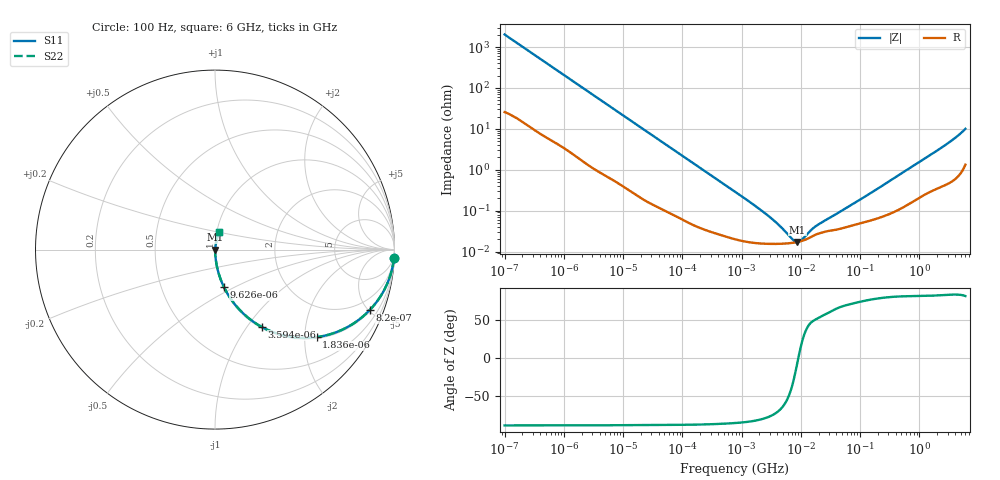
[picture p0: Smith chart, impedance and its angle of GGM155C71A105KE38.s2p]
!Murata Part Number: GGM155C71A105KE38
!These Parameters are Measured in Series Mode Connection
!Data Generated on Jun 19, 2026
!  o--ll--o
!Port1  Port2
!  o------o
!Operation Temp=25[degC], DC Bias Voltage=0[V]
!Freq. Start=100[Hz] Stop=6[GHz] 401[Steps]
# Hz S RI R 50
!Freq.(Hz) S11(Real) S11(Imag) S21(Real) S21(Imag) S12(Real) S12(Imag) S22(Real) S22(Imag)
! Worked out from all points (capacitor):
!   401 points, 100 Hz to 6 GHz, reference 50 ohm
!   read as one part in series: C = 778 nF near 109 Hz
!   lowest |Z| = 17.2 mohm at 8.692 MHz (marker M1)
!   series resonance near 9.067 MHz, so ESL is about 400 pH
!   S11 on the Smith chart (normalised r, x): 100 Hz: 2, -41; 820 Hz: 1.08, -5.07; 1.836 kHz: 1.04, -2.29; 3.594 kHz: 1.02, -1.18; 9.626 kHz: 1.01, -0.44; 6 GHz: 1.03, +0.20
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100  0.997 -0.0489  0.00302 0.0489  0.00302 0.0489  0.997 -0.0489
293  0.9783 -0.1388  0.0217 0.1388  0.0217 0.1388  0.9783 -0.1388
524  0.9367 -0.2361  0.0633 0.2361  0.0633 0.2361  0.9367 -0.2361
820  0.8615 -0.3375  0.1385 0.3375  0.1385 0.3375  0.8615 -0.3375
1174  0.7566 -0.4211  0.2434 0.4211  0.2434 0.4211  0.7566 -0.4211
1836  0.5655 -0.4877  0.4345 0.4877  0.4345 0.4877  0.5655 -0.4877
2008  0.5222 -0.4916  0.4778 0.4916  0.4778 0.4916  0.5222 -0.4916
3594  0.26 -0.4307  0.74 0.4307  0.74 0.4307  0.26 -0.4307
5625  0.1288 -0.3264  0.8712 0.3264  0.8712 0.3264  0.1288 -0.3264
9626  0.0504 -0.2098  0.9496 0.2098  0.9496 0.2098  0.0504 -0.2098
18841  0.0149 -0.1122  0.9851 0.1122  0.9851 0.1122  0.0149 -0.1122
40335  0.00404 -0.0535  0.996 0.0535  0.996 0.0535  0.00404 -0.0535
774597  0.000208 -0.0029  0.9998 0.0029  0.9998 0.0029  0.000208 -0.0029
2837864  0.000154 -0.000726  0.9998 0.000726  0.9998 0.000726  0.000154 -0.000726
4440638  0.000154 -0.000391  0.9998 0.000391  0.9998 0.000391  0.000154 -0.000391
7266822  0.000163 -0.000112  0.9998 0.000112  0.9998 0.000112  0.000163 -0.000112
8692127  0.00017 -2.12e-05  0.9998 2.12e-05  0.9998 2.12e-05  0.00017 -2.12e-05
1.039699e7  0.000181 6.84e-05  0.9998 -6.84e-05  0.9998 -6.84e-05  0.000181 6.84e-05
1.555665e7  0.000235 0.000265  0.9998 -0.000265  0.9998 -0.000265  0.000235 0.000265
3.124326e8  0.00085 0.00518  0.9992 -0.00518  0.9992 -0.00518  0.00085 0.00518
2.450438e9  0.00515 0.0353  0.9949 -0.0353  0.9949 -0.0353  0.00515 0.0353
6e9  0.0225 0.0959  0.9775 -0.0959  0.9775 -0.0959  0.0225 0.0959
